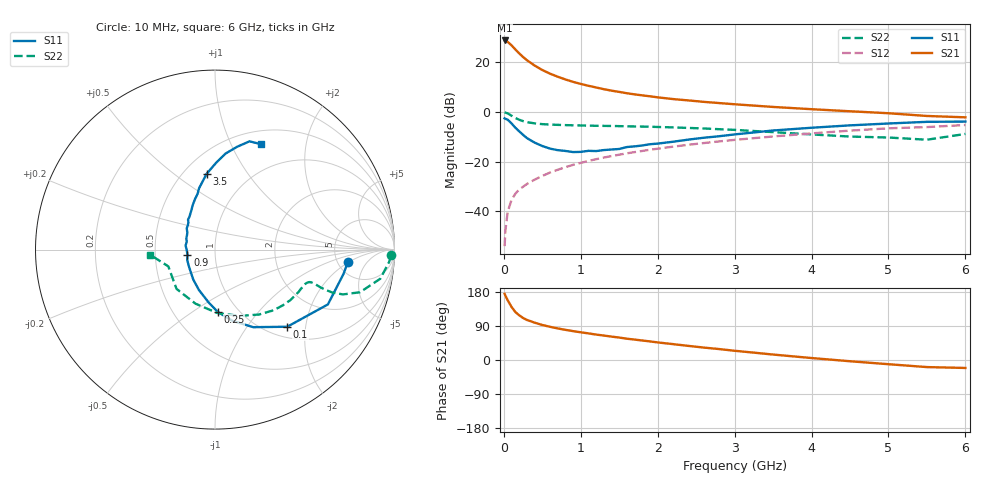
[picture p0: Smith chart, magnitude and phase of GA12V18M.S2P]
! Infineon Technologies  Discrete & RF Semiconductors
! BF775
! Si NPN RF Bipolar Junction Transistor in SOT23
! VCE = 12 V  IC = 18 mA
! Common Emitter S-Parameters:  May  1996
# GHz  S  MA  R  50
!  f  S11  S21  S12  S22
! GHz  MAG  ANG  MAG  ANG  MAG  ANG  MAG  ANG
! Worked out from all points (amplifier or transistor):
!   36 points, 10 MHz to 6 GHz, reference 50 ohm
!   highest |S21| = 28.8 dB at 10 MHz (marker M1)
!   |S21| within 3 dB of that: start of sweep to 131.2 MHz
!   unconditionally stable (mu >= 1): 485.7 MHz to 2.614 GHz
!   at 250 MHz: K = 0.78, MSG = 26.1 dB, |S12| = -30.1 dB
!   at 1.4 GHz: K = 1.09, MAG = 11.3 dB, |S12| = -17.7 dB
!   at 6 GHz: K = 0.87, MSG = 1.5 dB, |S12| = -5.2 dB
!   S11 on the Smith chart (normalised r, x): 10 MHz: 6.23, -1.88; 100 MHz: 1.21, -1.59; 250 MHz: 0.81, -0.64; 900 MHz: 0.73, -0.04; 3.5 GHz: 0.64, +0.66; 6 GHz: 0.66, +1.31
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0.01  0.7439 -5.2  27.43 174.6  0.002 87.6  0.9826 -1.9
0.02  0.7288 -10.7  27.14 170.0  0.0041 82.5  0.9717 -4.2
0.05  0.6992 -25.9  25.69 157.6  0.0098 75.9  0.9351 -10.0
0.1  0.5887 -46.9  21.87 140.1  0.0171 70.4  0.842 -16.4
0.15  0.4817 -63.8  18.07 126.5  0.0227 65.9  0.7555 -19.3
0.2  0.408 -76.4  15.08 117.9  0.0277 65.5  0.6969 -20.1
0.25  0.3469 -87.5  12.74 110.9  0.0313 65.0  0.6543 -20.0
0.3  0.2985 -96.5  11 105.7  0.0356 66.3  0.6244 -19.7
0.4  0.2422 -111.7  8.588 98.6  0.0435 67.4  0.5901 -19.0
0.5  0.2065 -125.8  6.974 92.4  0.0517 68.6  0.5691 -18.8
0.6  0.1833 -137.9  5.9 87.6  0.0605 69.0  0.5587 -18.9
0.7  0.1707 -150.1  5.12 83.4  0.0687 69.8  0.5503 -19.3
0.9  0.1561 -169.2  4.031 76.2  0.0864 69.3  0.5388 -20.7
1.1  0.1653 172.1  3.362 70.2  0.1037 68.9  0.5308 -23.1
1.3  0.1714 158.9  2.87 64.5  0.1212 67.6  0.5247 -25.3
1.6  0.1973 142.9  2.38 56.2  0.1475 65.7  0.5141 -29.5
2.2  0.252 121.9  1.817 41.9  0.2006 61.0  0.4895 -39.3
2.6  0.3033 111.5  1.597 32.8  0.2371 57.4  0.4657 -47.0
3.5  0.424 96.4  1.262 14.4  0.3215 47.8  0.3932 -69.9
4.5  0.5378 83.8  1.033 -3.3  0.4215 35.8  0.3202 -109.9
5.5  0.6332 72.3  0.831 -18.7  0.4967 20.2  0.2765 -160.3
6  0.6408 66.4  0.78 -21.0  0.5467 15.8  0.3614 -175.3
